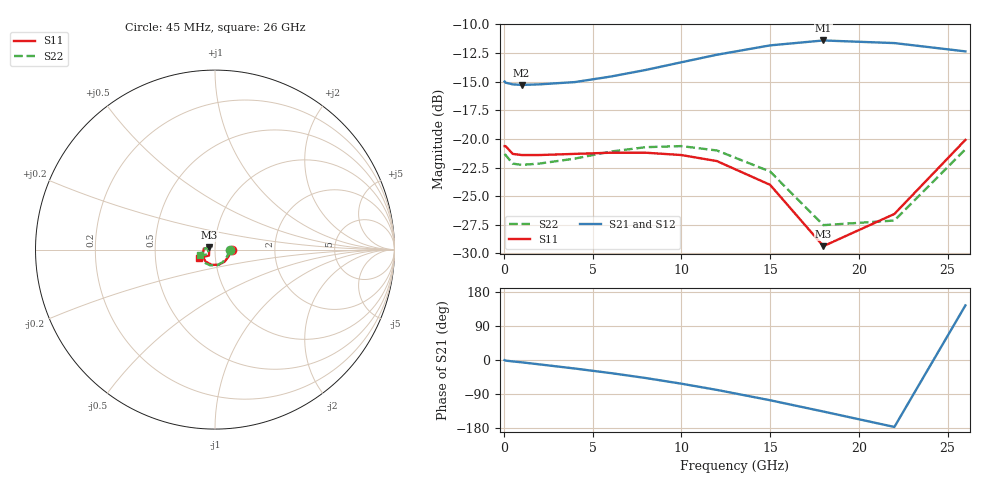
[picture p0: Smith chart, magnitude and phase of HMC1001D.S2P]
! HMMC-1001
! Typical s-parameters at 15dB attenuation setting, TA = 25 C
# ghz s ma r 50
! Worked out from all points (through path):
!   14 points, 45 MHz to 26 GHz, reference 50 ohm
!   highest |S21| = -11.40 dB at 18 GHz (marker M1); lowest = -15.3 dB at 1 GHz (marker M2)
!   lowest |S11| = -29.4 dB at 18 GHz (marker M3), VSWR 1.07, Z = 46.9 + j1.11 ohm
!   |S11| at or under -10 dB: start of sweep to end of sweep
!   |S22| runs from -27.5 to -20.6 dB; largest |S21 - S12| = 0.0059
0.045  0.093 -1.3  0.178 -0.4  0.178 -0.7  0.086 -2.2
0.1  0.093 -3.7  0.176 -1.6  0.176 -1.6  0.085 -4.5
0.5  0.086 -8.3  0.173 -3.7  0.172 -3.5  0.078 -9.2
1  0.085 -13.6  0.172 -6.1  0.171 -6.0  0.077 -15.7
2  0.085 -25.8  0.173 -11.5  0.172 -11.4  0.078 -29.5
4  0.086 -51.2  0.177 -22.5  0.177 -22.5  0.082 -57.0
6  0.087 -76.5  0.187 -34.4  0.188 -34.4  0.088 -82.0
8  0.087 -101.6  0.2 -47.6  0.2 -47.7  0.092 -105.9
10  0.085 -126.9  0.216 -62.5  0.217 -62.6  0.093 -128.4
12  0.08 -151.6  0.233 -78.9  0.234 -78.8  0.089 -150.3
15  0.063 175.0  0.256 -106.2  0.256 -106.3  0.072 -179.4
18  0.034 159.6  0.269 -136.0  0.268 -136.1  0.042 164.8
22  0.047 -135.5  0.262 -176.7  0.264 -176.7  0.044 -144.1
26  0.099 -151.7  0.241 144.0  0.241 142.6  0.09 -159.5
